{attribute 'GUID' := '56AA2C33-D736-E752-6308-29B40FF3D0B1'}
TYPE DUT_BalluffSmartLight :
	STRUCT
		 {attribute 'GUID' := '56AA2C34-D736-E752-6308-29B40FF3D0B1'}
		In AT %I* : DUT_BalluffSmartLightIn;
		 {attribute 'GUID' := '56AA2C35-D736-E752-6308-29B40FF3D0B1'}
		Out AT %Q* : DUT_BalluffSmartLightOut;
	END_STRUCT
END_TYPE
